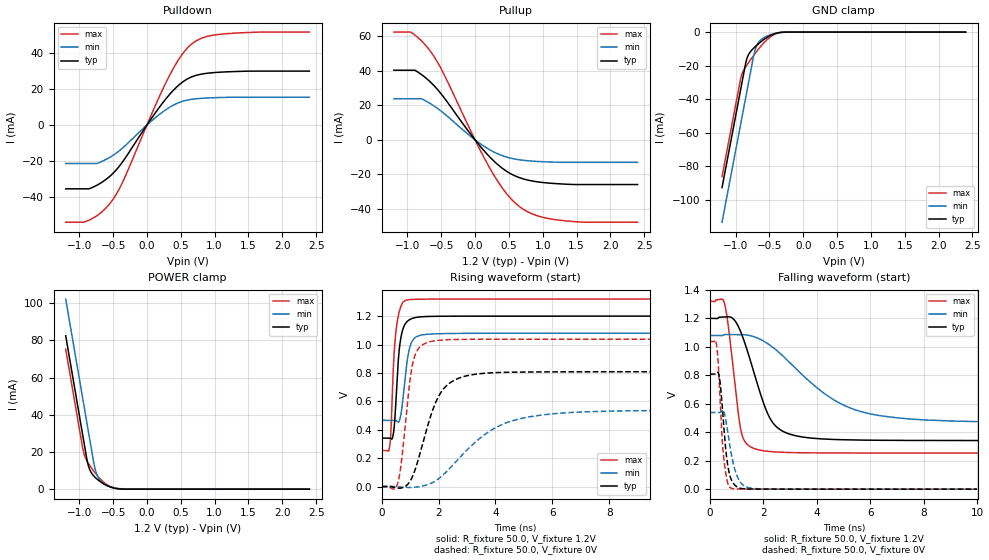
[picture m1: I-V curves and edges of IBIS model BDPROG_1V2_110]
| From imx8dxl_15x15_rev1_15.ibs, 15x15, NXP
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[Model] BDPROG_1V2_110
Model_type I/O
Polarity   Non-Inverting
Enable   Active-Low
| CAP_THRESHOLD on pad IO is "CMOS" :
| Rising=10.0% of vdde1v2   Falling=90.0% of vdde1v2
| C_comp min and max val. don't necessarily correlate with the min and max pvt
| but are the smallest and greatest pad capacitance found.
| var   typ   min   max
C_comp   2.02665pF  2.00435pF  2.04880pF
Vinl = 324.0mV
Vinh = 924.0mV
Vmeas = 600.0mV   | Reference voltage for timing measurements
Cref  = 15.0pF   | Timing specification test load capacitance value
Rref  = 1.0MOhm   | Timing specification test load resistance value
Vref  = 1.2V   | Timing specification test load voltage
[Model Spec]
| TIME_THRESHOLD on pin ZI is "CORE" :
| Rising=50.0% of vdd   Falling=50.0% of vdd
Vinl 420.00000mV 378.00000mV 462.00000mV
Vinh 780.00000mV 702.00000mV 858.00000mV
| variable   typ   min   max
[Temperature Range] 25.0 125.0 -40.0
| variable   typ   min   max
[Voltage Range] 1.2V 1.08V 1.32V
| variable   typ   min   max
[POWER Clamp Reference] 1.2V 1.08V 1.32V
| variable   typ   min   max
[GND Clamp Reference] 0V 0V 0V
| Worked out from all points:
|   slope of the pulldown table from 0 to 0.18 V, typ, clamps not added: 18.8 ohm
|   slope of the pullup table from 0 to 0.18 V, typ, clamps not added: 21.5 ohm
|   GND clamp passes 1 mA (typ) near -0.42 V on its own axis
|   POWER clamp passes 1 mA (typ) near -0.53 V on its own axis
|   rising waveform, R_fixture 50.0, V_fixture 1.2V: 20-80 % time 183ps typ, 228ps min, 168ps max; typ from 0.342 V to 1.2 V
|   falling waveform, R_fixture 50.0, V_fixture 1.2V: 20-80 % time 902ps typ, 2.41ns min, 395ps max; typ from 1.2 V to 0.342 V
|   rising waveform, R_fixture 50.0, V_fixture 0V: 20-80 % time 788ps typ, 1.87ns min, 342ps max; typ from 0 V to 0.808 V
|   falling waveform, R_fixture 50.0, V_fixture 0V: 20-80 % time 239ps typ, 344ps min, 196ps max; typ from 0.808 V to 0 V
[POWER Clamp]
-1.2V     82.47mA    102.2mA    75.29mA
-950mV    29.35mA    49.08mA    22.16mA
-920mV    22.97mA    42.71mA    17.94mA
-870mV    13.26mA    32.08mA    14.19mA
-830mV    9.388mA    23.58mA    11.94mA
-790mV    7.28mA     15.08mA    9.891mA
-760mV    6.153mA    10.18mA    8.467mA
-710mV    4.618mA    5.741mA    6.312mA
-650mV    3.105mA    3.261mA    4.124mA
-520mV    918uA      1.114mA    1.041mA
-370mV    66.09uA    190.5uA    36.14uA
2.4V      0A         0A         0A
[GND Clamp]
-1.2V     -92.79mA   -113.4mA   -86.23mA
-920mV    -33.29mA   -53.93mA   -27.01mA
-890mV    -26.92mA   -47.56mA   -23.57mA
-840mV    -16.83mA   -36.93mA   -20.11mA
-800mV    -12.88mA   -28.43mA   -17.73mA
-720mV    -9.099mA   -11.98mA   -13.24mA
-680mV    -7.622mA   -7.471mA   -11.12mA
-620mV    -5.599mA   -4.428mA   -8.161mA
-470mV    -1.717mA   -1.41mA    -2.413mA
-410mV    -792.7uA   -748.8uA   -1.042mA
-300mV    -72.27uA   -128.2uA   -61.83uA
2.4V      12.46nA    838.5nA    861.8pA
| variable   typ   min   max
[Pullup Reference] 1.2V 1.08V 1.32V
| variable   typ   min   max
[Pulldown Reference] 0V 0V 0V
[Pullup]
-1.2V     40.43mA    23.85mA    62.55mA
-950mV    40.43mA    23.85mA    62.55mA
-790mV    37.84mA    23.85mA    57.37mA
-650mV    33.18mA    20.76mA    50.85mA
-480mV    25.62mA    15.99mA    39.67mA
-70mV     3.554mA    2.169mA    5.679mA
210mV     -9.632mA   -5.605mA   -15.89mA
440mV     -17.55mA   -9.676mA   -29.96mA
660mV     -21.99mA   -11.59mA   -38.82mA
890mV     -24.18mA   -12.44mA   -43.65mA
1.2V      -25.4mA    -12.94mA   -46.37mA
2.4V      -25.92mA   -13.04mA   -47.77mA
[Pulldown]
-1.2V     -35.25mA   -21.25mA   -53.68mA
-850mV    -35.2mA    -21.25mA   -52.48mA
-690mV    -32.22mA   -20.51mA   -48.75mA
-510mV    -27.02mA   -16.97mA   -41.49mA
-350mV    -19.86mA   -12.39mA   -30.83mA
100mV     5.438mA    3.275mA    8.68mA
320mV     16.23mA    9.427mA    26.34mA
520mV     23.53mA    13mA       38.97mA
680mV     26.84mA    14.29mA    45.29mA
830mV     28.26mA    14.8mA     48.26mA
1.11V     29.23mA    15.21mA    50.22mA
2.4V      29.76mA    15.37mA    51.31mA
[Ramp]
dV/dt_r 484.94348mV/788.01804ps 322.86552mV/1.86938ns 622.7264mV/342.04065ps
dV/dt_f 515.05443mV/901.65758ps 368.20966mV/2.41473ns 639.70262mV/394.82486ps
R_load = 50.0
| Removed startup time: 0s 0s 0s  .
| Removed end time: 10.0ns.
[Rising Waveform]
R_fixture   = 50.0
V_fixture   = 1.2V
V_fixture_min = 1.08V
V_fixture_max = 1.32V
0s        341.6mV    466.3mV    253.8mV
282ps     341.8mV    466.3mV    284.1mV
330ps     337.8mV    466.3mV    408.7mV
400ps     360.2mV    466.3mV    791mV
488ps     555.8mV    466.7mV    1.068V
618ps     964.8mV    460.6mV    1.231V
810ps     1.139V     740.5mV    1.308V
1.026ns   1.18V      1.004V     1.317V
1.42ns    1.196V     1.067V     1.319V
10ns      1.2V       1.08V      1.32V
| Removed startup time: 0s 0s 0s  .
| Removed end time: 50.0ns.
[Falling Waveform]
R_fixture   = 50.0
V_fixture   = 1.2V
V_fixture_min = 1.08V
V_fixture_max = 1.32V
0s        1.2V       1.08V      1.32V
560ps     1.21V      1.086V     1.296V
710ps     1.211V     1.086V     1.119V
1.09ns    1.134V     1.086V     497mV
1.24ns    1.064V     1.085V     361.9mV
2.12ns    550.2mV    1.028V     266.7mV
2.9ns     392.6mV    905.7mV    257.7mV
4.96ns    347.4mV    594.7mV    254.1mV
7.98ns    342.1mV    486.8mV    253.8mV
50ns      341.6mV    466.3mV    253.8mV
| Removed startup time: 0s 0s 0s  .
| Removed end time: 50.0ns.
[Rising Waveform]
R_fixture   = 50.0
V_fixture   = 0V
V_fixture_min = 0V
V_fixture_max = 0V
0s        7.051nV    441.6nV    4.403nV
580ps     -11.43mV   -200.8uV   35.1mV
710ps     -8.88mV    -3.855mV   201.9mV
1.01ns    41.38mV    -6.789mV   771.6mV
1.18ns    121.4mV    -4.175mV   928.3mV
1.97ns    623.6mV    50.71mV    1.029V
2.67ns    759.8mV    188.4mV    1.036V
4.13ns    803.1mV    427.5mV    1.038V
6.92ns    807.9mV    524.7mV    1.038V
50ns      808.2mV    538.1mV    1.038V
| Removed startup time: 0s 0s 0s  .
| Removed end time: 10.0ns.
[Falling Waveform]
R_fixture   = 50.0
V_fixture   = 0V
V_fixture_min = 0V
V_fixture_max = 0V
0s        808.2mV    538.1mV    1.038V
226ps     807.9mV    538.1mV    1.041V
342ps     801.7mV    537.8mV    790.1mV
440ps     638.2mV    549mV      412.9mV
518ps     445.5mV    550.3mV    222.9mV
644ps     201.4mV    432.4mV    62.81mV
782ps     77.06mV    268.5mV    7.898mV
1.096ns   8.907mV    61.87mV    883.9uV
1.526ns   1.024mV    7.595mV    339.7uV
10ns      645.6nV    12.43uV    63.78nV
